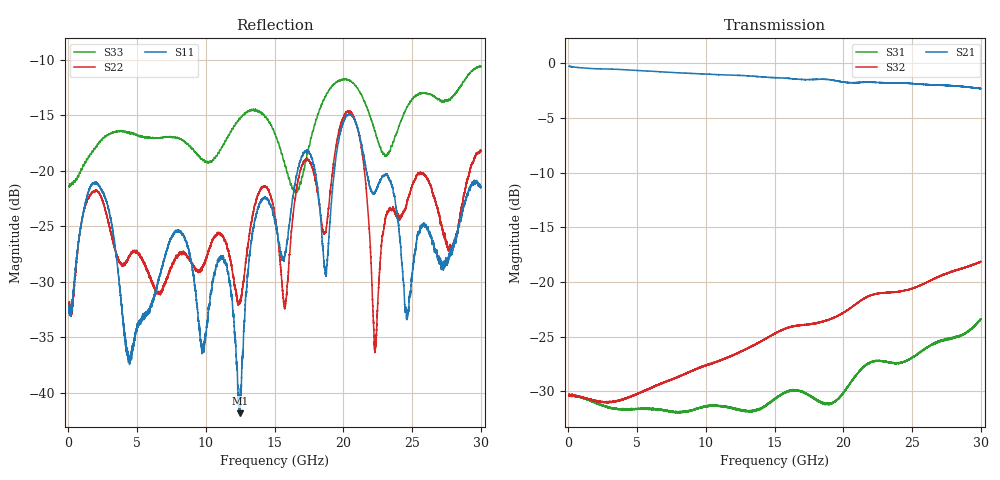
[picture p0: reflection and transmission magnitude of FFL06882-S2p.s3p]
!The following data was pulled from an Agilent PNA
!This sNp file was generated from the data in the RF Test software
!NOTE:  Smoothing/Math/Corrections applied on any given trace ARE included in the data saved here
# MHz S dB R 50
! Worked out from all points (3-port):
!   12801 points, 50 MHz to 30 GHz, reference 50 ohm
!   strongest paths, dB at 50 MHz, 7.537 GHz, 15.03 GHz, 22.51 GHz, 30 GHz:
!     S21: -0.3, -0.8, -1.3, -1.8, -2.3
!     S32: -30.4, -28.9, -24.7, -21.1, -18.1
!     S31: -30.3, -31.9, -30.7, -27.2, -23.4
!   lowest |S11| = -41.8 dB at 12.47 GHz (marker M1), VSWR 1.02, Z = 50.5 - j0.638 ohm
!   |S11| at or under -10 dB: start of sweep to end of sweep
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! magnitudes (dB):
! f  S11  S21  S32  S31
! 50 MHz  -32.3  -0.3  -30.4  -30.3
! 2.037 GHz  -21.1  -0.5  -30.9  -31.1
! 4.367 GHz  -37.3  -0.6  -30.6  -31.7
! 8.052 GHz  -25.4  -0.9  -28.7  -31.9
! 12.47 GHz  -41.8  -1.1  -26.4  -31.7
! 15.03 GHz  -24.6  -1.3  -24.7  -30.7
! 20.59 GHz  -15.0  -1.8  -22.3  -29.1
! 22.31 GHz  -21.9  -1.7  -21.1  -27.2
! 24.61 GHz  -33.1  -1.8  -20.7  -27.2
! 30 GHz  -21.5  -2.3  -18.1  -23.4
